// Demo接口
INTERFACE I_ShowMotion EXTENDS I_Base

PROPERTY P_Reset : BOOL
GET
END_GET
SET
END_SET
END_PROPERTY

// 如果为TRUE，启动运行
PROPERTY P_Start : BOOL
GET
END_GET
SET
END_SET
END_PROPERTY

// 如果为TRUE，则停止运动
PROPERTY P_Stop : BOOL
GET
END_GET
SET
END_SET
END_PROPERTY

// 运动模式
PROPERTY ShowPattern : INT
GET
END_GET
SET
END_SET
END_PROPERTY

END_INTERFACE
